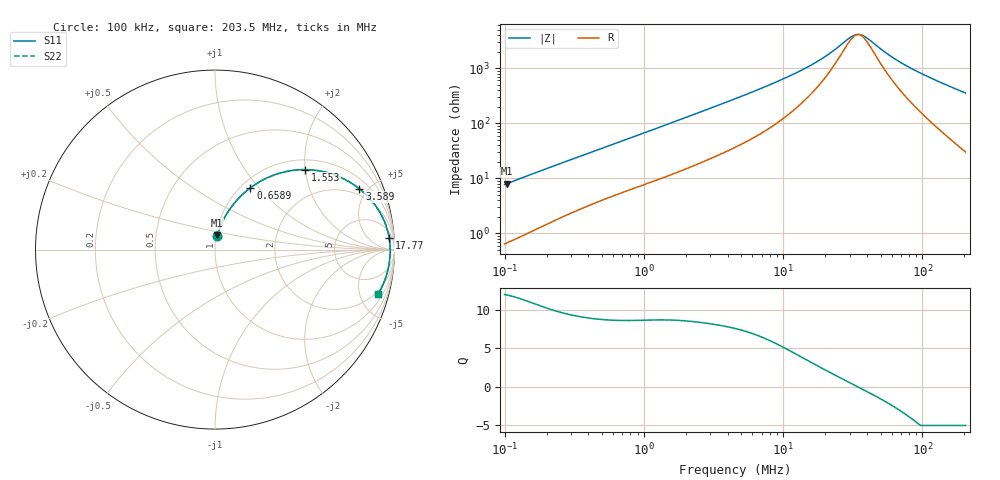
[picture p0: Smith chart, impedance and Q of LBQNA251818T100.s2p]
! LBQNA251818T100  S-PARAMETER MODEL  ( General Type )
! Model Generated by TAIYO YUDEN Corporation (http://www.ty-top.com)
! Version 1.0
! TAIYO YUDEN Control No. 191025NI43SB-FBB
! Copyright(c) 2019 TAIYO YUDEN CO.,LTD. All Rights Reserved.
! Product Description (link to TY-COMPAS)
! https://ds.yuden.co.jp/TYCOMPAS/or/detail?pn=LBQNA251818T100K&u=M
! Products Name : Inductors
! Characteristics :
!  Inductance : 10 uH , SRF(min) : 30 MHz , DC Resistance(max) : 0.325 Ohm
!  Rated Current : Saturation :250 mA , Temp Rise : 600 mA (20 degC)
!  Case Size : 2.5 x 1.8 / 0.098 x 0.071 [mm/inch] , Thickness : 1.8 / 0.071 [mm/inch]
!  (Conditions: Temperature = 25 degC , DC Bias Current/Voltage = 0A / 0V)
! External Node Assignments :
!  1  o---GGG---o  2
! GND o---------o GND
! Frequency Range : 0.1MHz  -  203.457813MHz  [ 402 STEP ]
# MHz S RI R 50
! Freq[MHz].  S11 Real  S11 Imag  S21 Real  S21 Imag  S12 Real  S12 Imag  S22 Real  S22 Imag
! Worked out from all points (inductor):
!   401 points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, 100 kHz to 203.5 MHz, reference 50 ohm
!   read as one part in series: L = 12.2 uH near 103.9 kHz
!   highest Q = 11.9 at 103.9 kHz (marker M1), where L = 12.3 uH
!   self-resonance near 34.51 MHz
!   S11 on the Smith chart (normalised r, x): 100 kHz: 1.01, +0.15; 658.9 kHz: 1.10, +0.90; 1.553 MHz: 1.23, +2.00; 3.589 MHz: 1.56, +4.42; 17.77 MHz: 10, +25; 203.5 MHz: 1.61, -7.08
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0.1  0.0122 0.0758  0.9878 -0.0758  0.9878 -0.0758  0.0122 0.0758
0.103882  0.0129 0.0786  0.9871 -0.0786  0.9871 -0.0786  0.0129 0.0786
0.194756  0.034 0.139  0.966 -0.139  0.966 -0.139  0.034 0.139
0.358236  0.0848 0.2288  0.9152 -0.2288  0.9152 -0.2288  0.0848 0.2288
0.658942  0.1968 0.3438  0.8032 -0.3438  0.8032 -0.3438  0.1968 0.3438
1.283332  0.4232 0.4398  0.5768 -0.4398  0.5768 -0.4398  0.4232 0.4398
1.552569  0.5028 0.4456  0.4972 -0.4456  0.4972 -0.4456  0.5028 0.4456
2.272346  0.6578 0.419  0.3422 -0.419  0.3422 -0.419  0.6578 0.419
3.589078  0.8042 0.3389  0.1958 -0.3389  0.1958 -0.3389  0.8042 0.3389
4.51063  0.8562 0.2911  0.1438 -0.2911  0.1438 -0.2911  0.8562 0.2911
9.125802  0.9442 0.1561  0.0558 -0.1561  0.0558 -0.1561  0.9442 0.1561
16.15871  0.9684 0.0768  0.0316 -0.0768  0.0316 -0.0768  0.9684 0.0768
17.77307  0.9704 0.0659  0.0296 -0.0659  0.0296 -0.0659  0.9704 0.0659
22.33659  0.9737 0.0417  0.0263 -0.0417  0.0263 -0.0417  0.9737 0.0417
30.29394  0.9759 0.0122  0.0241 -0.0122  0.0241 -0.0122  0.9759 0.0122
33.96119  0.9762 0.00149  0.0238 -0.00149  0.0238 -0.00149  0.9762 0.00149
36.64946  0.9763 -0.00563  0.0237 0.00563  0.0237 0.00563  0.9763 -0.00563
39.55054  0.9762 -0.0128  0.0238 0.0128  0.0238 0.0128  0.9762 -0.0128
57.88634  0.9739 -0.0504  0.0261 0.0504  0.0261 0.0504  0.9739 -0.0504
74.14835  0.9703 -0.0781  0.0297 0.0781  0.0297 0.0781  0.9703 -0.0781
98.6664  0.9628 -0.1156  0.0372 0.1156  0.0372 0.1156  0.9628 -0.1156
203.4578  0.9084 -0.2489  0.0916 0.2489  0.0916 0.2489  0.9084 -0.2489
